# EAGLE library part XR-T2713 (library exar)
LOOPBACK DETECTOR
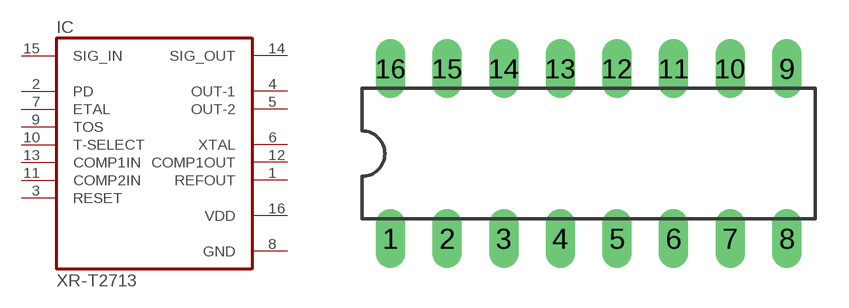
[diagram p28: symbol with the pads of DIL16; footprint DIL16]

Designator prefix IC

## XR-T2713 (OC_FARNELL: unknown; OC_NEWARK: unknown)  [DIL16]
1  REFOUT  out
2  PD  in
3  RESET  in
4  OUT-1  out
5  OUT-2  out
6  XTAL  out
7  ETAL  in
8  GND  pwr
9  TOS  in
10  T-SELECT  in
11  COMP2IN  in
12  COMP1OUT  out
13  COMP1IN  in
14  SIG_OUT  out
15  SIG_IN  in
16  VDD  pwr

## Footprint DIL16 (pad centres in mm)
Dual In Line Package
drill 0.813 long: 1 -8.89,-3.81; 2 -6.35,-3.81; 3 -3.81,-3.81; 4 -1.27,-3.81; 5 1.27,-3.81; 6 3.81,-3.81; 7 6.35,-3.81; 8 8.89,-3.81; 9 8.89,3.81; 10 6.35,3.81; 11 3.81,3.81; 12 1.27,3.81; 13 -1.27,3.81; 14 -3.81,3.81; 15 -6.35,3.81; 16 -8.89,3.81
